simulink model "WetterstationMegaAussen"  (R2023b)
settings: Solver=FixedStepDiscrete  StartTime=0.0  StopTime=Inf  FixedStep=0.01  RelTol=1e-3
libraries: arduinolib x1, arduinosensorlib x1, Arduino_Additional_Lib x1

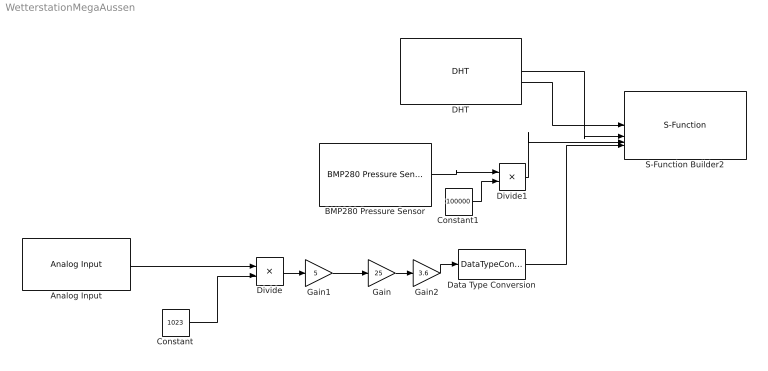
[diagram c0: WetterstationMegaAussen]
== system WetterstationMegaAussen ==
  Analog Input : arduinolib/Analog Input  pinNumber=1  ReadResultsOnly=off  ConversionTriggerSource=Software  ExternalTriggerType=uint32( 0 )  OutputDataType=uint16  EnableConversionCompleteNotify=off  EnableOuputStatus=off  SampleTime=-1  blockPlatform=arduino
  BMP280 Pressure Sensor : arduinosensorlib/BMP280 Pressure Sensor  I2CAddress=0x76  BitRate=1000000  IsActivePressure=on  IsActiveTemperature=off  IsStatus=off  FilterMode=0  PressureSensitivityFactor=2.62  TemperatureSensitivityFactor=0.005  DataType=double  SampleTime=-1
  Constant : Constant  Value=1023
  Constant1 : Constant  Value=100000
  DHT : Arduino_Additional_Lib/DHT  F=off  Pin=54  Tp=22  Ts=3
  Data Type Conversion : DataTypeConversion
  Divide : Product  Inputs=*/
  Divide1 : Product  Inputs=*/
  Gain : Gain  Gain=25
  Gain1 : Gain  Gain=5
  Gain2 : Gain  Gain=3.6
  S-Function Builder2 : S-Function  FunctionName=nRF24L01  SFunctionModules=nRF24L01_wrapper.cpp  SFunctionDeploymentMode=off  EnableBusSupport=off  mask(S-Function Builder){}
      mask help: Simulink:masks:SFunctionBuilder_MD
      mask init:
      | val = [[.9  0.75 0.75 1 1 .9 .9 1]',[1 1 0.75 0.75 .9 .9 1 .9]'];try , sys = get_param(gcb,'SfunBuilderFcnName');if isempty(sys), sys = get_param(gcb,'FunctionName'); end,catch, sys = get_param(gcb,'FunctionName'); end
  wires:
  DHT/1 -> S-Function Builder2/2
  DHT/2 -> S-Function Builder2/1
  Analog Input/1 -> Divide/1
  Data Type Conversion/1 -> S-Function Builder2/4
  Constant/1 -> Divide/2
  Divide/1 -> Gain1/1
  Gain1/1 -> Gain/1
  Gain/1 -> Gain2/1
  Gain2/1 -> Data Type Conversion/1
  Divide1/1 -> S-Function Builder2/3
  BMP280 Pressure Sensor/1 -> Divide1/1
  Constant1/1 -> Divide1/2
